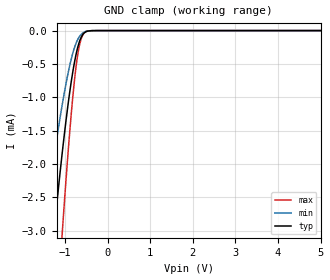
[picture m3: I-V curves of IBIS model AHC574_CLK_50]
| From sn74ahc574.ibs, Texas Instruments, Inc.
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[Model]   AHC574_CLK_50
Model_type  Input
Vinl = 1.65
Vinh = 3.85
| variable   typ   min   max
C_comp   0.91pF   0.77pF   1.07pF
[Temperature Range]   40   100   -40
| Ambient temperature   25   85   -40
[Voltage range]   5   4.5   5.5
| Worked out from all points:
|   GND clamp passes 1 mA (typ) near -0.91 V on its own axis
[GND Clamp]
| AHC574_CLK_50
|   Voltage   I(typ)   I(min)   I(max)
-5V       -39.31mA   -25.9mA    -50.38mA
-1.5V     -4.713mA   -3.008mA   -7.461mA
-1.27V    -3.094mA   -1.943mA   -5.031mA
-1.245V   -2.93mA    -1.835mA   -4.777mA
-1.07V    -1.855mA   -1.126mA   -3.072mA
-1.05V    -1.741mA   -1.051mA   -2.887mA
-875mV    -855.1uA   -481.5uA   -1.403mA
-765mV    -430.2uA   -230.1uA   -666.2uA
-665mV    -170.7uA   -92.15uA   -230.5uA
-615mV    -91.95uA   -52.33uA   -111.9uA
-545mV    -32.01uA   -20.15uA   -32.39uA
5V        14.69nA    957pA      135.7nA
